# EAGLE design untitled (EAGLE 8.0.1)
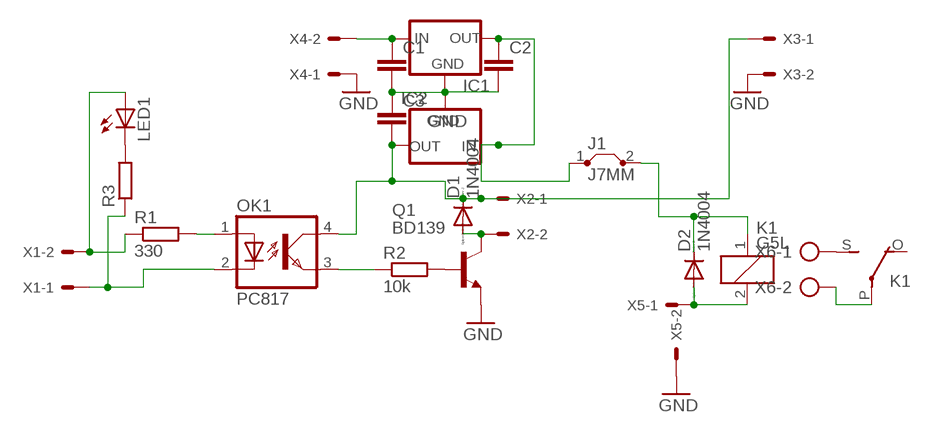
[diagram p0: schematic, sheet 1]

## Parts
C1  C-EU050-024X044  [C050-024X044]
C2  C-EU050-024X044  [C050-024X044]
C3  C-EU050-024X044  [C050-024X044]
D1  1N4004  [DO41-10]
D2  1N4004  [DO41-10]
IC1  78XXL  [78XXL]
IC2  78XXL  [78XXL]
J1  J7MM  [07]
K1  G5L  [G5LE]
LED1  LED3MM  [LED3MM]
OK1  PC817  [DIL04]
Q1  BD139  [TO126]
R1  330  R-EU_0207/7  [0207/7]
R2  10k  R-EU_0207/7  [0207/7]
R3  R-EU_0207/2V  [0207/2V]
X1  KK-156-2  [KK-156-2]
X2  KK-156-2  [KK-156-2]
X3  KK-156-2  [KK-156-2]
X4  KK-156-2  [KK-156-2]
X5  KK-156-2  [KK-156-2]
X6  AK300/2  [AK300/2]

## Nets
GND: C1.2 C2.2 C3.1 IC1.GND IC2.GND Q1.1(E) X3.2 X4.1 X5.2
N$1: LED1.A R1.1 X1.2
N$2: OK1.1(A) R1.2
N$3: OK1.2(C) R3.1 X1.1
N$4: Q1.3(B) R2.2
N$5: OK1.3(EMIT) R2.1
N$6: D1.A Q1.2(C) X2.2
N$8: C1.1 IC1.IN X4.2
N$10: C2.1 IC1.OUT IC2.IN J1.1
N$12: D2.A K1.2 X5.1
N$13: K1.S(2:S) X6.1
N$14: K1.P(2:P) X6.2
N$18: D2.C J1.2 K1.1
N$55: C3.2 D1.C IC2.OUT OK1.4(COL) X2.1 X3.1
N$59: LED1.K(C) R3.2
Unconnected: K1.O(2:O)

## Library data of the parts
C1-C3 = resistor:C-EU: CAPACITOR, European symbol
D1 D2 = diode:1N4004: DIODE
IC1 IC2 = v-reg:78XXL: VOLTAGE REGULATOR
J1 = jumper:J: Bridge
K1 = relay:G5L: RELAY 1 x switch, 10 A/120 V AC, 8 A/30 V ADC, Omron; OC_FARNELL: unknown; OC_NEWARK: unknown
LED1 = led:LED: LED
OK1 = optocoupler:PC817: SHARP OPTO COUPLER; MPN: PC817X4J000F; OC_FARNELL: 9707727; OC_NEWARK: 97K7059
Q1 = transistor-npn:BD139*: NPN Transistor
R1-R3 = resistor:R-EU_: RESISTOR, European symbol
X1-X5 = con-molex:KK-156-2: KK 156 HEADER; OC_FARNELL: unknown; OC_NEWARK: unknown
X6 = con-ptr500:AK300/2: CONNECTOR; OC_FARNELL: unknown; OC_NEWARK: unknown

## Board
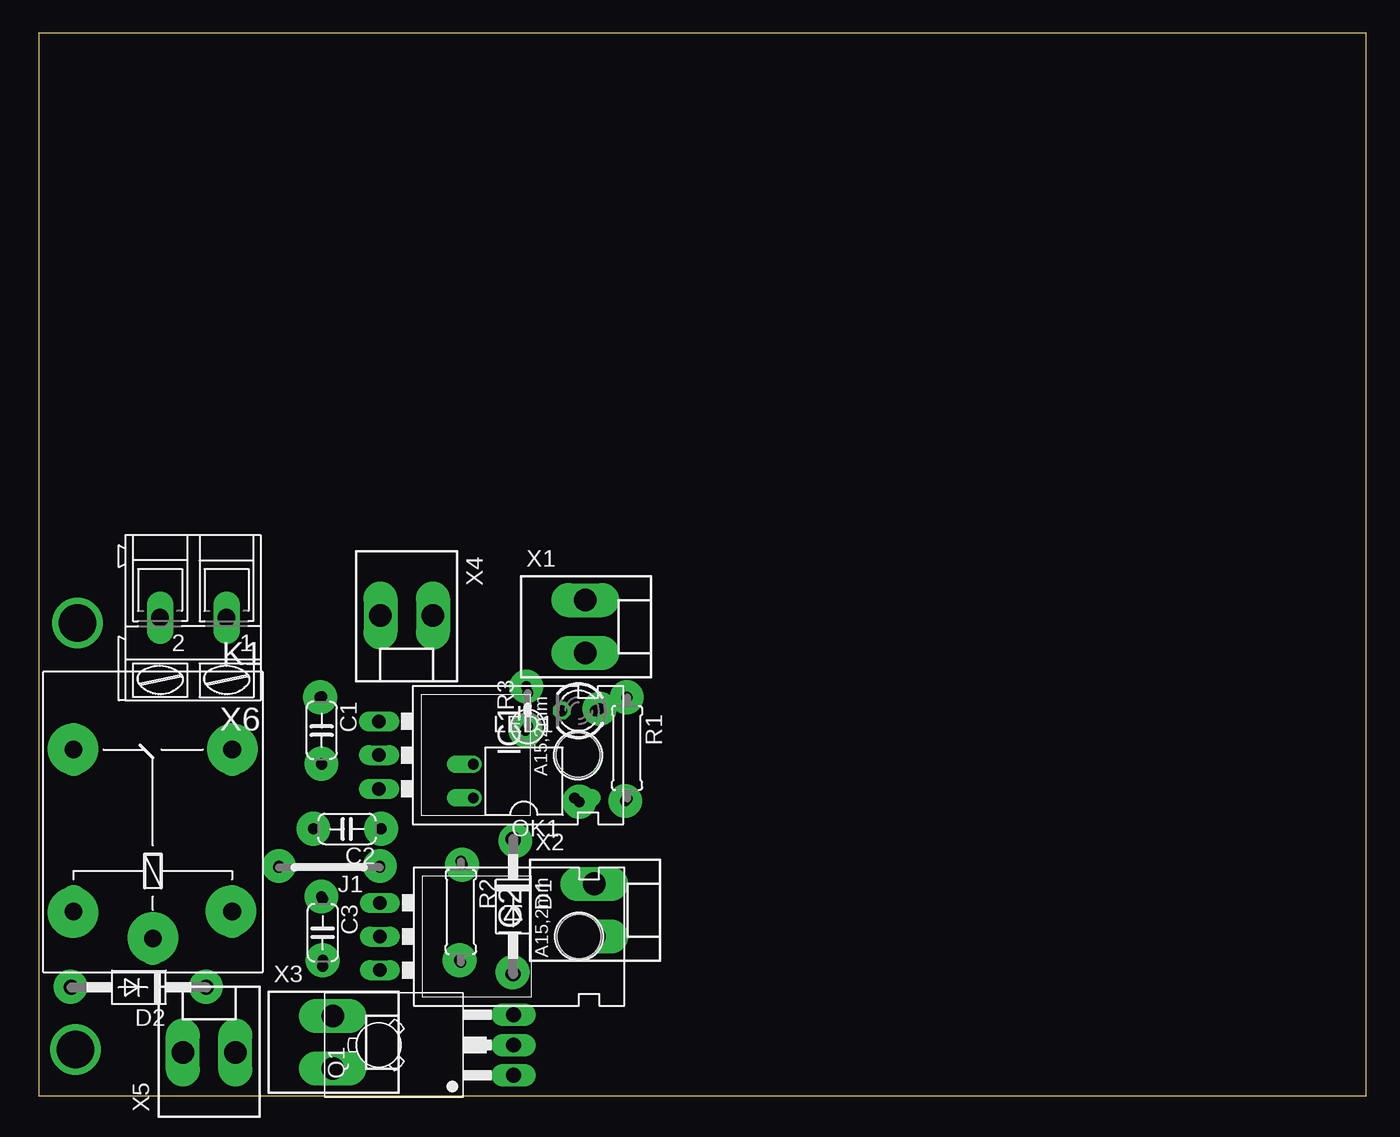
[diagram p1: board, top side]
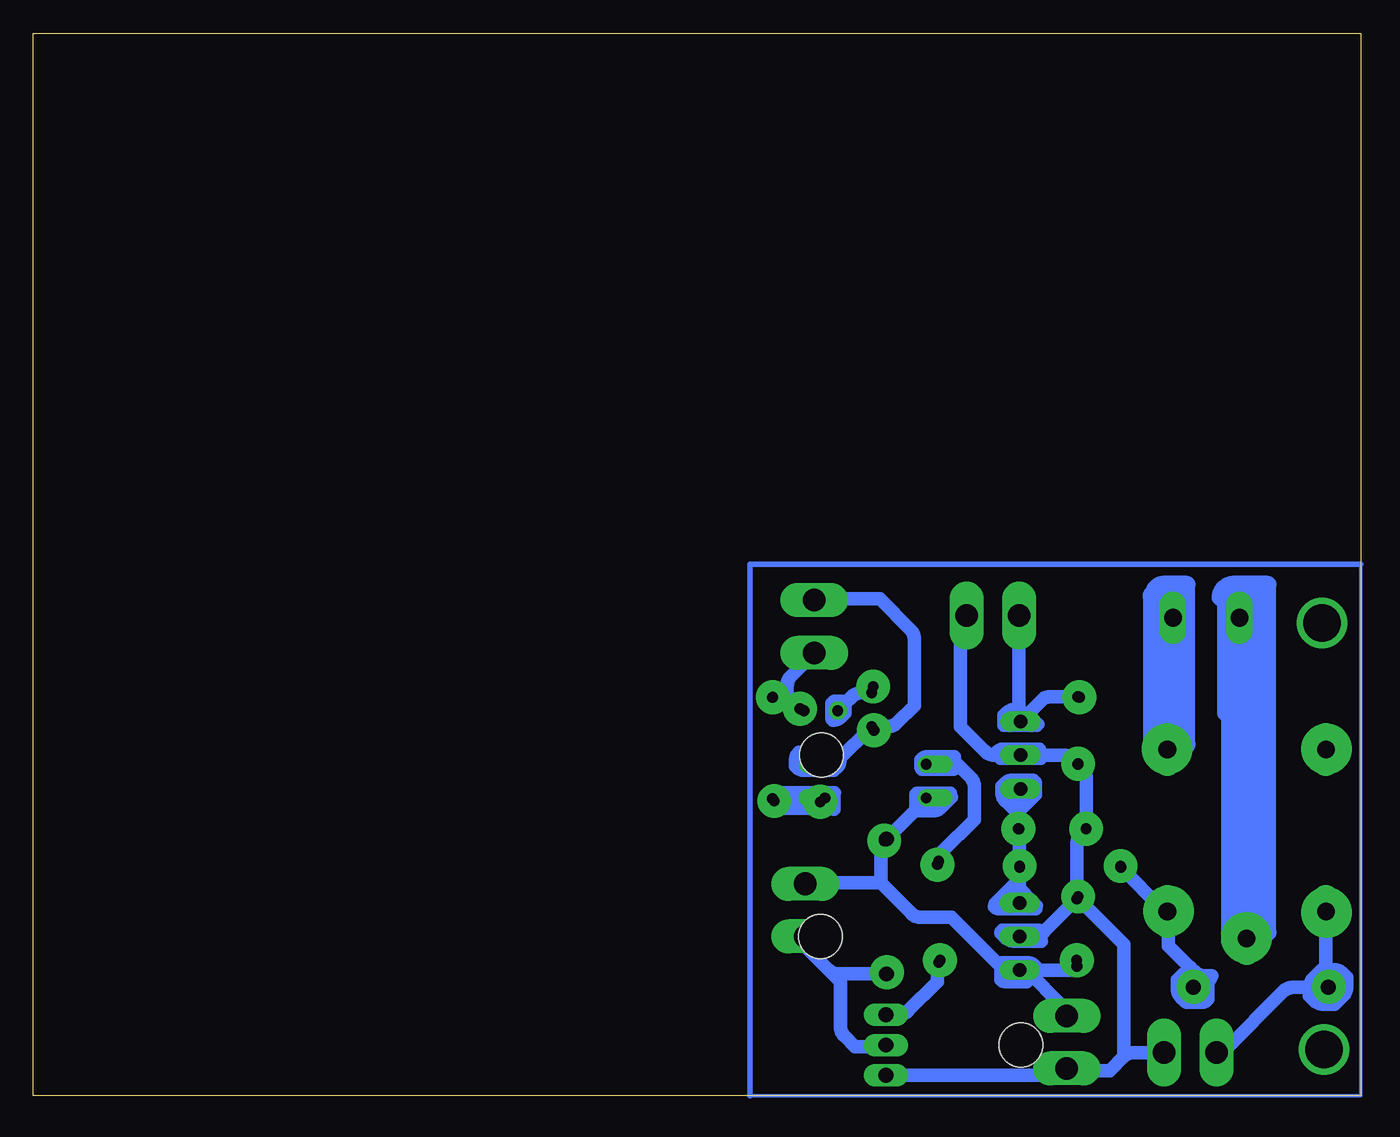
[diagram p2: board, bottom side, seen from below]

Size 100 x 80 mm. Coordinates in mm from the lower left corner, seen from the top.
Outline: 0,0 100,0 100,80 0,80 0,0
Copper layers (1*16): Top 0.035mm / dielectric 1.5mm / Bottom 0.035mm
Design rules "default": minimum track width 10mil, minimum drill 24mil, track to track 8mil, track to pad 8mil, pad to pad 8mil, via to via 8mil, smd to smd 8mil, copper to edge 40mil, drill to drill 8mil, minimum pad ring 10mil, minimum via ring 8mil, stop-mask expansion 4mil, vias tented up to drill 0mil, thermal gap 10mil

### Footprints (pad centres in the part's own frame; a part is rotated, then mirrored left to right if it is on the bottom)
C050-024X044 = drill 0.813 octagon: 1 -2.54,0; 2 2.54,0
DO41-10 = drill 1.118: A 5.08,0; C -5.08,0
78XXL = drill 1.016 long: GND 0,-3.81; IN -2.54,-3.81; OUT 2.54,-3.81 | hole 3.302: 0,11.176
07 = drill 0.813 pad 1.6 octagon: 1 -3.81,0; 2 3.81,0
G5LE = drill 1.321 long: 1 -7.493,-5.969; 2 -7.493,5.969; O 4.699,5.969; P -9.525,0; S 4.699,-5.969
LED3MM = drill 0.813 octagon: A -1.27,0; K 1.27,0
DIL04 = drill 0.813 offset: 1 -1.27,-3.81; 2 1.27,-3.81; 3 1.27,3.81; 4 -1.27,3.81
TO126 = drill 1.118 long: 1 -2.286,-5.08; 2 0,-5.08; 3 2.286,-5.08 | hole 3.302: 0,5.08
0207/7 = drill 0.813 octagon: 1 -3.81,0; 2 3.81,0
0207/2V = drill 0.813 octagon: 1 -1.27,0; 2 1.27,0
KK-156-2 = drill 1.7 pad 2.184 long: 1 -1.98,0; 2 1.98,0
AK300/2 = drill 1.321 long: 1 -2.515,0; 2 2.489,0

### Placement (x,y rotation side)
C1  21.32,27.51 270 top
C2  23.23,20.08 180 top
C3  21.4,12.28 270 top
D1  35.74,14.25 270 top
D2  7.55,8.16 180 top
IC1  29.45,25.65 270 top
IC2  29.52,11.99 270 top
J1  21.9,17.2 180 top
K1  8.61,21.37 90 top
LED1  40.67,28.99 180 top
OK1  36.55,23.69 90 top
Q1  30.69,3.82 90 top
R1  44.32,26.18 270 top
R2  31.8,13.84 270 top
R3  36.84,29.07 90 top
X1  41.17,35.33 270 top
X2  41.85,13.98 270 top
X3  22.15,4.04 270 top
X4  27.73,36.17 180 top
X5  12.84,3.25 0 top
X6  11.64,35.99 180 top

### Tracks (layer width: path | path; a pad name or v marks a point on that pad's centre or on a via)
GND
  Bottom 1.016: X5.2 17.14,3.25 arc-45 17.84,2.96 | 17.84,2.96 18.9,1.9 21.76,1.9 arc45 X3.2 arc90 22.68,1.53 Q1.1 | C3.1 21.4,18.96 arc90 21.38,18.98 arc45 21.09,19.68 C2.2 20.69,23.93 arc-45 20.98,24.63 C1.2 21.71,25.36 arc-45 22.41,25.65 IC1.GND 27.62,25.65 arc45 28.32,25.94 30.15,27.77 30.15,35.32 arc45 29.86,36.02 X4.1 | IC2.GND 24.64,11.99 arc-45 23.94,12.28 C3.1 | C3.1 arc45 21.21,14.74 17.87,11.4 17.87,3.02 arc-45 17.84,2.96
N$1
  Bottom 1.016: X1.2 42.92,31.6 arc-45 43.21,30.9 43.21,29.49 | 43.21,29.49 43,29.28 arc-45 42.3,28.99 LED1.A | R1.1 44.11,29.78 arc-45 43.41,29.49 43.21,29.49
N$2
  Bottom 1.016: R1.2 40.48,22.37 arc-45 OK1.1
N$3
  Bottom 1.016: OK1.2 40.09,24.96 arc-45 39.39,25.25 R3.1 35.63,27.8 arc-45 34.93,28.09 33.64,29.38 33.64,34.4 arc-45 33.93,35.1 36.24,37.41 40.93,37.41 arc-45 X1.1
N$4
  Bottom 1.016: Q1.3 34.81,6.11 arc-45 34.1,6.4 31.9,8.6 31.9,9.79 arc45 R2.2
N$5
  Bottom 1.016: R2.1 31.8,17.69 arc45 31.51,18.39 29.11,20.79 29.11,23.26 arc-45 29.4,23.96 30.51,25.07 32.47,25.07 arc-45 OK1.3
N$6
  Bottom 1.016: X2.2 41.85,11.66 arc-45 41.56,10.96 40.85,10.25 | 40.85,10.25 39.2,8.6 39.2,5.21 arc-45 38.91,4.51 38.1,3.7 36.06,3.7 arc-45 Q1.2 | D1.A 39.36,9.17 arc45 40.06,9.46 40.85,10.25
N$7  (via drill 2.8 pad 3.81)
  other vias: 2.93,35.6
N$8
  Bottom 1.016: X4.2 25.75,28.46 arc-45 IC1.IN 24.07,29.76 arc45 23.37,30.05 C1.1
N$9
  Bottom 1.016: 30.62,25.52 32.62,25.52 arc-45 33.15,25.3 33.15,24.84 arc-45 33.05,24.6 30.69,24.6 arc-45 30.59,24.64
N$10
  Bottom 1.016: 26,23.26 arc45 IC1.OUT arc-45 25.77,22.8 C2.1 arc45 25.71,19.93 J1.1 IC2.IN
N$11
  Bottom 0.254: 0.1,40 arc90 0,39.9 0,0 46,0
  Bottom 0.406: 0,40 0.1,40 46,40 46,0
N$12
  Bottom 1.016: K1.2 2.64,8.57 arc-45 D2.A 5.13,8.16 arc-45 5.83,7.87 10.3,3.4 10.5,3.4 arc-45 X5.1
N$13
  Bottom 1.016: K1.S 14.45,26.2 arc-45 14.15,26.91 X6.1
N$14
  Bottom 1.016: K1.P 8.61,35.03 arc-45 8.9,35.74 X6.2
N$15
  Bottom 1.016: 30.91,22.78 33.33,22.78 arc-45 33.5,22.71 33.5,21.52 arc45 33.53,21.45 32.27,21.45 arc-45 31.57,21.74 30.85,22.46
N$16  (via drill 2.8 pad 3.81)
  other vias: 2.78,3.48
N$17
  Bottom 1.016: 31.63,22.21 31.92,22.21 arc-45 32.62,21.92 32.68,21.86
N$18
  Bottom 1.016: D2.C 12.63,9.02 arc-45 12.92,9.72 14.5,11.3 14.5,13.69 arc-45 K1.1 arc45 14.9,14.01 J1.2
N$20  (via drill 0.8 pad 2.54)
  other vias: 21.2,30
N$21  (via drill 0.8 pad 2.54)
  other vias: 44.3,30
N$22  (via drill 0.8 pad 2.54)
  other vias: 42.25,29.14
N$23  (via drill 0.8 pad 2.54)
  other vias: 44.18,22.19
N$24  (via drill 0.8 pad 2.54)
  other vias: 36.68,27.52
N$25  (via drill 0.8 pad 2.54)
  other vias: 40.73,22.13
N$26  (via drill 0.8 pad 2.54)
  other vias: 36.74,30.81
N$27  (via drill 0.8 pad 2.54)
  other vias: 21.3,25
N$28  (via drill 0.8 pad 2.54)
  other vias: 20.7,20.1
N$29  (via drill 0.8 pad 2.54)
  other vias: 21.3,15
N$30  (via drill 0.8 pad 2.54)
  other vias: 18.1,17.3
N$31  (via drill 0.8 pad 2.54)
  other vias: 12.6,8.2
N$32  (via drill 0.8 pad 2.54)
  other vias: 2.4,8.2
N$33  (via drill 0.8 pad 2.54)
  other vias: 21.4,10.2
N$34  (via drill 0.8 pad 2.54)
  other vias: 35.7,9.3
N$35  (via drill 0.8 pad 2.54)
  other vias: 31.7,10.2
N$36  (via drill 0.8 pad 2.54)
  other vias: 31.9,17.4
N$37  (via drill 0.8 pad 2.54)
  other vias: 35.9,19.2
N$38  (via drill 0.8 pad 2.54)
  other vias: 25.8,20.1
N$39  (via drill 0.8 pad 2.54)
  other vias: 25.7,17.3
N$40  (via drill 0.8 pad 3.81)
  other vias: 14.6,26.1
N$41  (via drill 0.8 pad 3.81)
  other vias: 2.6,26.1
N$42  (via drill 0.8 pad 3.81)
  other vias: 2.6,13.8
N$43  (via drill 0.8 pad 3.81)
  other vias: 8.6,11.9
N$44  (via drill 0.8 pad 3.81)
  other vias: 14.5,13.9
N$45
  Bottom 1.27: 7.8,12.2 arc90 7,12.3 7,38.5 9.6,38.5 arc-90 10.6,37.5 arc90 10.2,37.1 10.2,28.8 arc90 9.9,28.5 9.9,11.6 8.6,11.6 arc-90 7.6,12.6 7.6,12.9 arc90 8,13.3 8,37.5 8.9,37.5 arc90 9.5,38.1 arc90 9,37.6 9,12.6 arc-90 8.7,12.9 8.7,15.9
N$46
  Bottom 1.27: 13.2,38.5 14.9,38.5 arc-90 15.6,37.8 arc-90 15.8,37.6 15.8,25.9 13.7,25.9 arc-90 13.3,26.3 arc-90 13.1,26.5 13.1,38.5 arc-90 13.6,38 13.6,37.8 13.9,37.8 arc-90 14.9,36.8 14.9,26.3 14.8,26.3 arc-90 13.8,27.3 13.8,37
N$55
  Bottom 1.016: 25.17,9.45 IC2.OUT 26.45,9.45 arc45 27.15,9.74 30.85,13.44 33.16,13.44 arc45 33.86,13.73 36.15,16.02 | 25.17,9.45 22.1,9.45 arc-45 C3.2 | X3.1 arc-45 22.44,6.72 25.17,9.45 | 36.15,16.02 41.7,16.02 arc-45 X2.1 | 36.15,16.02 36.15,18.51 arc45 35.86,19.21 D1.C 32.8,22.27 arc-45 OK1.4
N$56
  Bottom 1.016: 39.79,24.49 41.85,24.49 arc45 42.55,24.78 42.59,24.82 42.59,25.18 arc45 42.31,25.86 40.19,25.86 arc45 39.49,25.57 39.23,25.31 arc45 39.49,24.68 39.68,24.49
N$57
  Bottom 1.016: 40.07,25.13 41.48,25.13 arc45 41.91,25.31
N$58
  Bottom 1.016: 39.65,22.83 43.94,22.83 arc-45 44.08,22.77 44.08,21.64 39.87,21.64 arc45 39.7,21.57 39.7,22.71 arc45 39.65,22.83
N$59
  Bottom 1.016: 39.26,29.38 arc45 39.13,29.69 39.12,29.7 39.53,29.7 arc-45 39.84,29.57 39.84,28.47 arc-45 39.76,28.28 arc-45 39.09,28.56 38.85,28.8 38.85,29.43 arc45 38.77,29.62 | LED1.K 38.77,29.62 | 38.77,29.62 38.34,30.05 arc45 37.64,30.34 R3.2 | 38.77,29.62 arc-45 39.42,29.35 39.55,29.22
N$60
  Bottom 1.016: 25.14,8.59 26.74,8.59 arc45 27.1,8.74 27.1,9.83 arc45 27.02,10.02 25.21,10.02 arc45 24.51,9.73 24.36,9.58
N$61
  Bottom 1.016: 24.05,11.64 26.1,11.64 arc45 26.8,11.93 27.11,12.24 arc45 27.04,12.41 26.99,12.46 24.38,12.46 arc45 23.9,12.26
N$62
  Bottom 1.016: 24.47,14.07 27.2,14.07 arc45 27.59,14.23 arc45 27.43,14.61 26.04,16 arc-45 25.99,15.88 24.43,14.32 25.24,14.32 arc45 25.94,14.61 26.24,14.91
N$63
  Bottom 1.016: 24.69,23.76 26.17,23.76 arc-45 26.87,23.47 27.04,23.3 27.04,22.86 arc-45 26.75,22.16 25.96,21.37 arc-45 25.67,21.49 24.5,22.66 24.5,23.41 arc-45 24.63,23.72 25.78,22.57 arc45 26.21,22.75 26.27,22.81 26.27,22.88 arc45 25.93,22.74 25.58,22.39
N$64
  Bottom 1.016: 24.2,26.1 26.88,26.1 arc-45 27.46,25.86 arc-45 27.35,25.59 27.17,25.41 24.19,25.41 arc-45 24.07,25.46
N$65
  Bottom 1.016: 25.74,29.08 26.03,29.08 arc-45 26.73,28.79 26.88,28.64 26.88,27.88 24.56,27.88 arc-45 24.32,27.98 arc45 24.59,28.09 25.19,28.69 25.79,28.69 arc-45 26.44,28.42
N$66
  Bottom 1.016: 2.36,9.5 2.07,9.5 arc45 1.37,9.21 1.07,8.91 1.07,8.19 arc45 1.36,7.49 1.95,6.9 2.84,6.9 arc45 3.54,7.19 3.88,7.53 3.88,8.13 arc45 3.59,8.83 2.98,9.44
N$67
  Bottom 1.016: 11.23,9.02 11.76,9.02 arc45 12.46,9.31 12.48,9.33 12.82,9.33 arc-45 13.52,9.04 13.84,8.72 13.84,8.12 arc-45 13.55,7.42 13.16,7.03 12.07,7.03 arc-45 11.54,7.25 11.54,8.29 arc45 11.3,8.87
